TYPE "ST_AcyclicWriteResponse"
VERSION : 0.1


  STRUCT
   byServiceID : BYTE ;	//Service ID | Service ID related to the request sent by the client
   dwMessageID : DWORD ;	//Message ID | Message ID related to the request sent by the client
   dwDataLength : DWORD ;	//Data length | Must be 0x04 in this response (Object index, Sub index, Data type
   byAcknowledge : BYTE ;	//Acknowledge | 0x00 if the access was OK or value unequal 0x00 if not | See ackn
   dwWriteType : DWORD ;	//Write type | Write type related to the request sent by the client
   wIndex : WORD ;	//Index | Index of the object to be written
   bySubIndex : BYTE ;	//Sub Index | Sub Index of the object to be written
   byDataType : BYTE ;	//Data type | Data type of the object to be written
  END_STRUCT ;
END_TYPE

